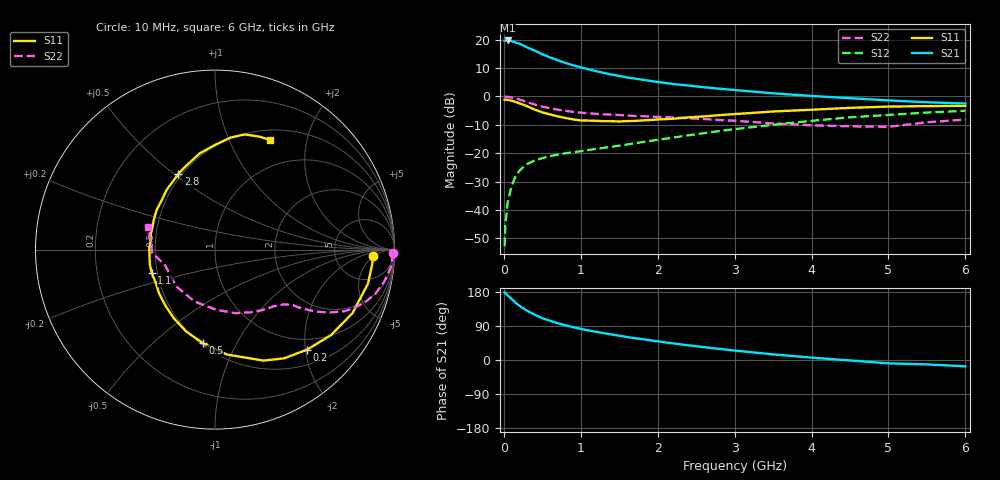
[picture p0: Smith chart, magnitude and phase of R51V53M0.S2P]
! SIEMENS Small Signal Semiconductors
! BFR183
! Si NPN RF Bipolar Junction Transistor in SOT23
! VCE = 1.5 V  IC = 3 mA
! Common Emitter S-Parameters:  May  1996
# GHz  S  MA  R  50
!  f  S11  S21  S12  S22
! GHz  MAG  ANG  MAG  ANG  MAG  ANG  MAG  ANG
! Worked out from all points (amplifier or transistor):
!   36 points, 10 MHz to 6 GHz, reference 50 ohm
!   highest |S21| = 19.7 dB at 50 MHz (marker M1)
!   |S21| within 3 dB of that: start of sweep to 351 MHz
!   unconditionally stable (mu >= 1): 1.228 GHz to 2.818 GHz
!   at 250 MHz: K = 0.30, MSG = 21.5 dB, |S12| = -24.9 dB
!   at 1.4 GHz: K = 1.05, MAG = 11.3 dB, |S12| = -17.8 dB
!   at 6 GHz: K = 0.92, MSG = 1.3 dB, |S12| = -5.0 dB
!   S11 on the Smith chart (normalised r, x): 10 MHz: 14, -5; 200 MHz: 0.78, -2.04; 500 MHz: 0.51, -0.74; 1.1 GHz: 0.47, -0.14; 2.8 GHz: 0.48, +0.52; 6 GHz: 0.62, +1.43
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0.01  0.879 -2.5  9.62 178.4  0.0023 87.7  0.994 -1.1
0.02  0.8802 -5.0  9.583 176.0  0.0054 88.6  0.9886 -2.2
0.05  0.8732 -12.5  9.701 170.4  0.0137 82.2  0.9855 -5.6
0.1  0.844 -24.8  9.426 161.2  0.0263 76.6  0.9594 -10.8
0.15  0.8032 -36.3  8.963 151.7  0.0384 70.7  0.9261 -15.5
0.2  0.7577 -47.3  8.545 143.7  0.0484 65.7  0.8832 -19.6
0.25  0.7182 -57.5  7.914 136.6  0.0566 61.1  0.8384 -22.9
0.3  0.6748 -66.4  7.358 130.2  0.064 58.0  0.7994 -25.4
0.4  0.5885 -83.5  6.428 119.6  0.0745 52.8  0.7226 -29.1
0.5  0.5246 -97.6  5.547 110.4  0.0818 49.8  0.6606 -31.5
0.6  0.483 -109.7  4.874 103.5  0.0888 48.1  0.6195 -32.9
0.7  0.4457 -121.1  4.354 97.2  0.0942 47.1  0.5865 -34.0
0.8  0.4171 -131.5  3.897 91.7  0.0995 46.7  0.559 -34.9
0.9  0.3951 -142.3  3.551 86.5  0.1043 47.2  0.5347 -35.4
1.1  0.3755 -159.8  3.01 78.2  0.1135 48.4  0.5054 -37.3
1.6  0.3681 166.2  2.164 60.6  0.1421 51.1  0.462 -42.8
2.2  0.4047 137.1  1.662 43.8  0.1885 53.0  0.4269 -52.4
2.8  0.4681 115.8  1.372 29.4  0.2454 51.0  0.3839 -66.1
3.5  0.5432 99.0  1.136 14.9  0.3166 44.8  0.3346 -89.3
4.5  0.6301 82.1  0.932 -1.2  0.429 32.7  0.2979 -136.8
5.5  0.6761 68.6  0.79 -11.6  0.5205 19.3  0.3505 -177.2
6  0.6835 63.3  0.751 -16.7  0.5595 10.8  0.3921 161.3
